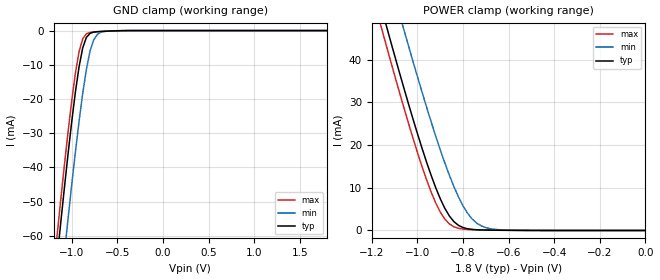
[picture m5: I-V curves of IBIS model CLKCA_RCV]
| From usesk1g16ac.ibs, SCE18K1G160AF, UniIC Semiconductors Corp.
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|   Model CLKCA_RCV
[Model]  CLKCA_RCV
Model_type Input
Polarity   Non-Inverting
Vinl = 360.000mV
Vinh = 1440.000mV
C_comp   0.9549pF   0.9383pF   0.9648pF
[Temperature Range]   25.0000   70.0000   0.0
[Voltage Range]   1.8000V   1.7000V   1.9000V
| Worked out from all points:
|   GND clamp passes 1 mA (typ) near -0.81 V on its own axis
|   POWER clamp passes 1 mA (typ) near -0.81 V on its own axis
[GND_clamp]
|Voltage   I(typ)   I(min)   I(max)
-1.8V     -245.8mA   -264.8mA   -239.4mA
-1.16V    -66.45mA   -85.98mA   -59.71mA
-1.12V    -55.99mA   -75.42mA   -49.29mA
-1.08V    -45.79mA   -65.03mA   -39.17mA
-1.04V    -35.93mA   -54.86mA   -29.48mA
-960mV    -17.97mA   -35.49mA   -12.43mA
-920mV    -10.58mA   -26.55mA   -6.156mA
-880mV    -5.084mA   -18.39mA   -2.409mA
-840mV    -2.012mA   -11.4mA    -951.3uA
-760mV    -458.7uA   -2.729mA   -401uA
-640mV    -199.4uA   -240.4uA   -221.5uA
1.8V      1.691nA    751.7pA    250.2pA
[POWER_clamp]
|Voltage   I(typ)   I(min)   I(max)
-1.8V     183.7mA    197.1mA    179.3mA
-1.16V    52.46mA    66.29mA    47.81mA
-1.14V    48.58mA    62.39mA    43.92mA
-1.12V    44.72mA    58.52mA    40.07mA
-1.06V    33.41mA    47.07mA    28.82mA
-980mV    19.25mA    32.39mA    14.96mA
-920mV    10.02mA    22.1mA     6.447mA
-880mV    5.191mA    15.81mA    2.658mA
-840mV    2.06mA     10.24mA    858.4uA
-760mV    247.9uA    2.684mA    178.4uA
-680mV    76.03uA    412.6uA    99.61uA
0V        1.691nA    238.1pA    351.1pA
